PROGRAM MAIN
VAR
	fb_recipemancommands:recipemancommands;//配方功能块
	f_trig_save,f_trig_load:f_trig;//用于触发保存/读取的下降沿功能块
	bsave,bload:BOOL;//保存，读取按钮
	recipedefinitionname:STRING:='BOX';//配方表名称
	sfilepath:STRING:='E:\recipefiles\box';//文件路径
	filename:STRING:='box1';//文件名
END_VAR

f_trig_save(CLK:= bsave, Q=> );
f_trig_load(CLK:= bload, Q=> );

IF f_trig_save.Q THEN
	fb_recipemancommands.CreateRecipe(RecipeDefinitionName:= recipedefinitionname, RecipeName:= 'parameter1');
	fb_recipemancommands.ReadAndSaveRecipeAs(RecipeDefinitionName:= recipedefinitionname, RecipeName:= 'parameter1',
	FileName:= concat(concat(concat(sfilepath,'\'),filename),'.txtrecipe'));
END_IF

IF f_trig_load.Q THEN
	fb_recipemancommands.CreateRecipe(RecipeDefinitionName:= recipedefinitionname, RecipeName:= 'parameter1');
	fb_recipemancommands.LoadFromAndWriteRecipe(RecipeDefinitionName:= recipedefinitionname, RecipeName:= 'parameter1',
	FileName:= concat(concat(concat(sfilepath,'\'),filename),'.txtrecipe'));
END_IF

END_PROGRAM
